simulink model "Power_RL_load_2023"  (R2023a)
settings: Solver=VariableStepAuto  StartTime=0.0  StopTime=0.1  MaxStep=1e-5  RelTol=1e-3
libraries: spsRMSLib x2, spsACVoltageSourceLib x1, spsCurrentMeasurementLib x1, spsGroundLib x1, spsPowerLib x1, spsSeriesRLCBranchLib x1, spsVoltageMeasurementLib x1, spspowerguiLib x1

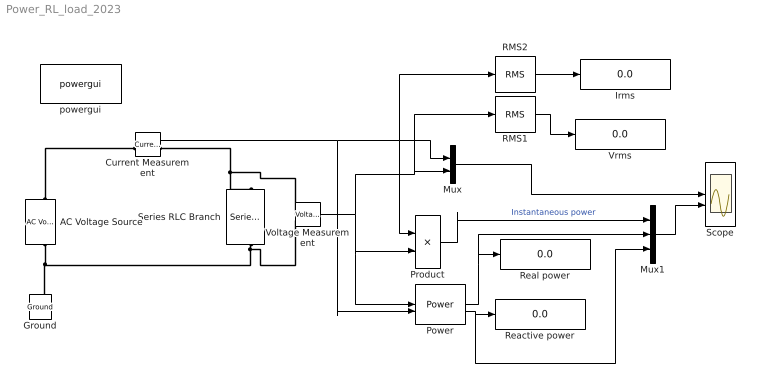
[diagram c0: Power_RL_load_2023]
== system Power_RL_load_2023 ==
  AC Voltage Source : spsACVoltageSourceLib/AC Voltage Source  Amplitude=100*sqrt(2)  Phase=0  Frequency=60  SampleTime=0  Measurements=None  BusType=swing  Pref=10e3  Qref=0  Qmin=-inf  Qmax=+inf
  Current Measurement : spsCurrentMeasurementLib/Current Measurement  PhasorSimulation=off  OutputType=Complex  PSBequivalent=0
  Ground : spsGroundLib/Ground  LConnTagsString=a
  Irms : Display
  Mux : Mux  Inputs=2
  Mux1 : Mux  Inputs=3
  Power : spsPowerLib/Power  Freq=60  Vinit=[1, 0]  Iinit=[1, 0]  Ts=0
  Product : Product
  RMS1 : spsRMSLib/RMS  TrueRMS=on  Freq=60  RMSInit=0  Ts=0
  RMS2 : spsRMSLib/RMS  TrueRMS=on  Freq=60  RMSInit=0  Ts=0
  Reactive power : Display
  Real power : Display
  Scope : Scope  NumInputPorts=2
  Series RLC Branch : spsSeriesRLCBranchLib/Series RLC Branch  LConnTagsString=__new0  RConnTagsString=__new0  BranchType=RL  Resistance=2  Inductance=5e-3  SetiL0=off  InitialCurrent=0  Capacitance=1e-6  Setx0=off  InitialVoltage=0  Measurements=None
  Voltage Measurement : spsVoltageMeasurementLib/Voltage Measurement  PhasorSimulation=off  OutputType=Complex  PSBequivalent=0
  Vrms : Display
  powergui : spspowerguiLib/powergui  Priority=1  SimulationMode=Continuous  SampleTime=50e-6  frequency=60  Iterations=50  frequencyindice=60  Pbase=100e6  ErrMax=1e-4  UnitsV=kV  UnitsW=MW  buscounter=0  FunctionMessages=off  echomessages=off  EnableUseOfTLC=off  CurrentSourceSwitches=off  DisableSnubberDevices=off  DisableRonSwitches=off  DisableVfSwitches=off  DisplayEquations=off  AutomaticDiscreteSolvers=off  SolverType=Tustin/Backward Euler (TBE)  Interpol=off  ExternalGateDelay=off  methode=off  Ts=100  x0status=blocks  SPID=on  SwTol=0  HookPort=off  NonlinearTolerance=1e-4  nMaxIteration=100  ContinueOnMaxIteration=off  RestoreLinks=warning  ResistiveCurrentMeasurement=off  Frange=[0:2:500]  Ylog=off  Xlog=on  ShowGrid=off  save=off  variable=ZData  structure=0  ZoomFFT=off  StartTime=0.0  cycles=1  DisplayStyle=1  fundamental=60  FreqAxis=off  MaxFrequency=1000  frequencyindicesteady=1  RmsSteady=1  display=off
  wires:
  Mux/1 -> Scope/1
  Voltage Measurement/1 -> Power/1, Product/2, RMS1/1, Mux/2
  Current Measurement/1 -> Power/2, RMS2/1, Product/1, Mux/1
  Power/1 -> Mux1/2, Real power/1
  Power/2 -> Mux1/3, Reactive power/1
  RMS2/1 -> Irms/1
  RMS1/1 -> Vrms/1
  Mux1/1 -> Scope/2
  Product/1 -> Mux1/1  "Instantaneous power"
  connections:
  Current Measurement/RConn1 -- Voltage Measurement/LConn1 -- Series RLC Branch/LConn1
  AC Voltage Source/RConn1 -- Current Measurement/LConn1
  AC Voltage Source/LConn1 -- Voltage Measurement/LConn2 -- Series RLC Branch/RConn1 -- Ground/LConn1
